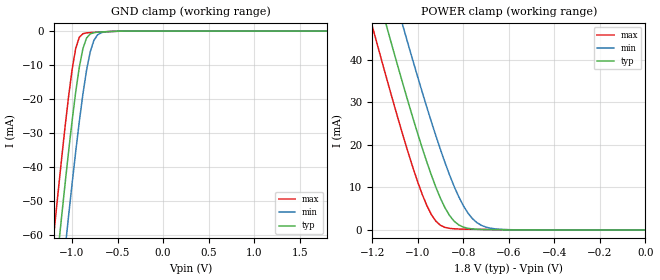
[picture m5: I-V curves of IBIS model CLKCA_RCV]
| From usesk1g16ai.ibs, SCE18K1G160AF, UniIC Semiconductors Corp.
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|   Model CLKCA_RCV
[Model]  CLKCA_RCV
Model_type Input
Polarity   Non-Inverting
Vinl = 360.000mV
Vinh = 1440.000mV
C_comp   0.9549pF   0.9383pF   0.9648pF
[Temperature Range]   25.0000   85.0000   -40.0000
[Voltage Range]   1.8000V   1.7000V   1.9000V
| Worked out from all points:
|   GND clamp passes 1 mA (typ) near -0.81 V on its own axis
|   POWER clamp passes 1 mA (typ) near -0.81 V on its own axis
[GND_clamp]
|Voltage   I(typ)   I(min)   I(max)
-1.8V     -245.8mA   -264.8mA   -229.4mA
-1.2V     -77.1mA    -96.68mA   -59.8mA
-1.16V    -66.45mA   -85.98mA   -49.22mA
-1.12V    -55.99mA   -75.42mA   -38.9mA
-1.08V    -45.79mA   -65.03mA   -28.98mA
-1.04V    -35.93mA   -54.86mA   -19.68mA
-960mV    -17.97mA   -35.49mA   -5.136mA
-880mV    -5.084mA   -18.39mA   -767.8uA
-800mV    -827.9uA   -6.067mA   -440uA
-760mV    -458.7uA   -2.729mA   -375.1uA
-680mV    -254.4uA   -478.8uA   -259.3uA
1.8V      1.691nA    751.7pA    225.3pA
[POWER_clamp]
|Voltage   I(typ)   I(min)   I(max)
-1.8V     183.7mA    197.1mA    172.1mA
-1.2V     60.32mA    74.16mA    48.04mA
-1.14V    48.58mA    62.39mA    36.32mA
-1.12V    44.72mA    58.52mA    32.49mA
-1.06V    33.41mA    47.07mA    21.39mA
-960mV    15.99mA    28.87mA    5.747mA
-900mV    7.429mA    18.88mA    1.096mA
-860mV    3.386mA    12.92mA    376uA
-800mV    675.4uA    5.743mA    195.2uA
-720mV    123.9uA    1.077mA    125.1uA
-600mV    29.78uA    68.1uA     52.6uA
0V        1.691nA    238.1pA    317.2pA
